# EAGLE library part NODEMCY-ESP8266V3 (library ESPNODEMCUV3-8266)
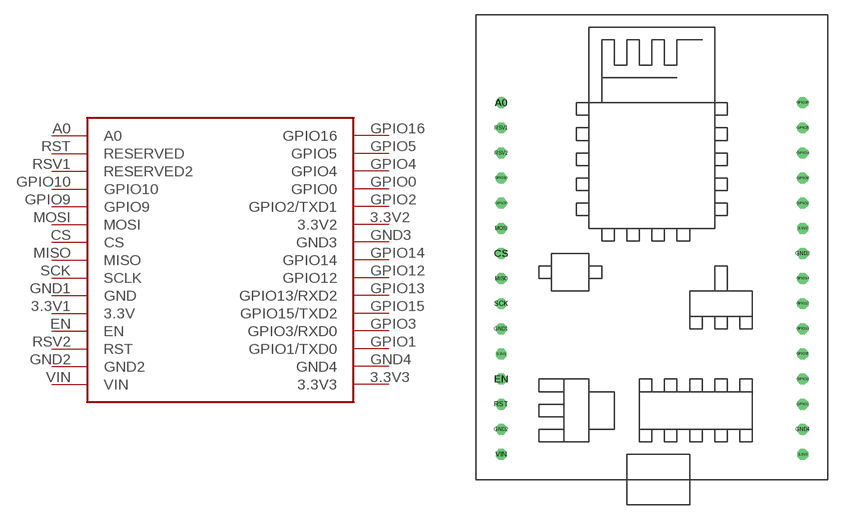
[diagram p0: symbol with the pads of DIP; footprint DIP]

Designator prefix -

## NODEMCY-ESP8266V3  [DIP]
3.3V1  3.3V
3.3V2  3.3V2
3.3V3  3.3V3
A0  A0
CS  CS
EN  EN
GND1  GND
GND2  GND2
GND3  GND3
GND4  GND4
GPIO0  GPIO0
GPIO1  GPIO1/TXD0
GPIO2  GPIO2/TXD1
GPIO3  GPIO3/RXD0
GPIO4  GPIO4
GPIO5  GPIO5
GPIO9  GPIO9
GPIO10  GPIO10
GPIO12  GPIO12
GPIO13  GPIO13/RXD2
GPIO14  GPIO14
GPIO15  GPIO15/TXD2
GPIO16  GPIO16
MISO  MISO
MOSI  MOSI
RST  RESERVED
RSV1  RESERVED2
RSV2  RST
SCK  SCLK
VIN  VIN

## Footprint DIP (pad centres in mm)
drill 0.6 octagon: 3.3V1 16.51,21.59; 3.3V2 46.99,34.29; 3.3V3 46.99,11.43; A0 16.51,46.99; CS 16.51,31.75; EN 16.51,19.05; GND1 16.51,24.13; GND2 16.51,13.97; GND3 46.99,31.75; GND4 46.99,13.97; GPIO0 46.99,39.37; GPIO1 46.99,16.51; GPIO2 46.99,36.83; GPIO3 46.99,19.05; GPIO4 46.99,41.91; GPIO5 46.99,44.45; GPIO9 16.51,36.83; GPIO10 16.51,39.37; GPIO12 46.99,26.67; GPIO13 46.99,24.13; GPIO14 46.99,29.21; GPIO15 46.99,21.59; GPIO16 46.99,46.99; MISO 16.51,29.21; MOSI 16.51,34.29; RST 16.51,16.51; RSV1 16.51,44.45; RSV2 16.51,41.91; SCK 16.51,26.67; VIN 16.51,11.43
